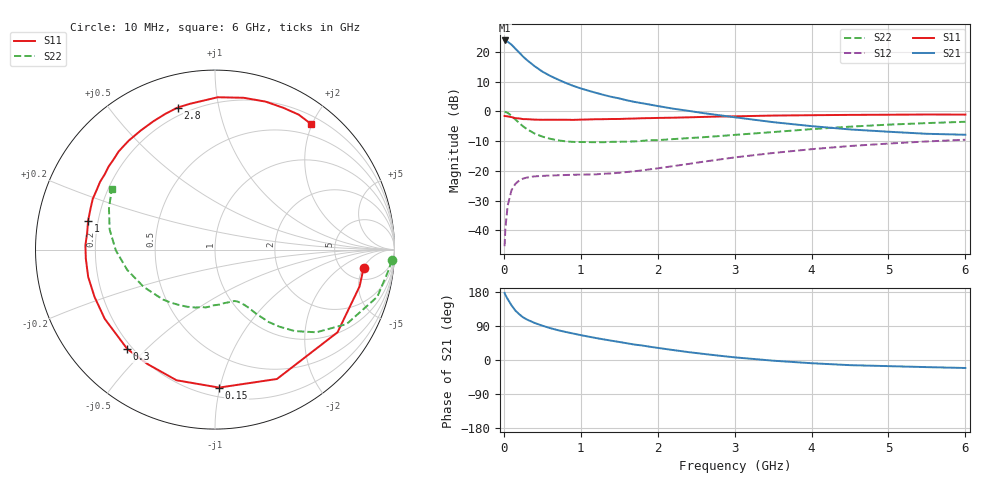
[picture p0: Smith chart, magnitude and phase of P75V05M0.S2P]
! SIEMENS Small Signal Semiconductors
! BFP196
! Si NPN RF Bipolar Junction Transistor in SOT143
! VCE = 5 V  IC = 5 mA
! Common Emitter S-Parameters:  May  1996
# GHz  S  MA  R  50
!  f  S11  S21  S12  S22
! GHz  MAG  ANG  MAG  ANG  MAG  ANG  MAG  ANG
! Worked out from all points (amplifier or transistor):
!   36 points, 10 MHz to 6 GHz, reference 50 ohm
!   highest |S21| = 23.8 dB at 10 MHz (marker M1)
!   |S21| within 3 dB of that: start of sweep to 159.2 MHz
!   unconditionally stable (mu >= 1): 1.146 GHz to 3.193 GHz
!   at 250 MHz: K = 0.25, MSG = 20.5 dB, |S12| = -22.6 dB
!   at 1.4 GHz: K = 1.14, MAG = 10.6 dB, |S12| = -20.9 dB
!   at 6 GHz: K = 0.99, MSG = 0.8 dB, |S12| = -9.6 dB
!   S11 on the Smith chart (normalised r, x): 10 MHz: 7.55, -5.13; 150 MHz: 0.26, -0.99; 300 MHz: 0.18, -0.44; 1 GHz: 0.16, +0.11; 2.8 GHz: 0.16, +0.76; 6 GHz: 0.32, +1.98
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0.01  0.8344 -7.1  15.56 177.0  0.0054 85.8  0.9867 -3.5
0.02  0.8312 -14.3  15.33 171.8  0.0108 84.6  0.9748 -6.6
0.05  0.8236 -34.0  14.78 160.7  0.0261 72.7  0.9419 -16.2
0.1  0.7993 -64.4  13.22 144.2  0.0474 58.5  0.8426 -29.5
0.15  0.7691 -88.3  11.33 130.4  0.0604 47.2  0.7289 -39.2
0.2  0.7589 -106.4  9.73 120.8  0.0687 39.9  0.6356 -45.6
0.25  0.7403 -120.6  8.328 112.7  0.0739 34.3  0.5598 -50.1
0.3  0.7385 -131.5  7.289 106.8  0.077 30.7  0.5029 -53.4
0.4  0.7254 -147.9  5.75 97.8  0.0806 25.9  0.4227 -57.4
0.5  0.7211 -158.6  4.668 90.6  0.0821 23.1  0.3759 -59.8
0.6  0.7228 -167.9  3.963 84.3  0.0832 22.1  0.346 -62.3
0.7  0.7214 -175.9  3.443 78.8  0.0841 21.6  0.3263 -64.7
0.8  0.7224 178.2  3.022 74.2  0.0849 21.6  0.3131 -67.1
1  0.7251 167.1  2.43 65.6  0.0861 23.0  0.3047 -71.6
1.1  0.7298 162.0  2.223 61.7  0.0867 24.2  0.3034 -74.4
1.6  0.7519 142.0  1.532 44.1  0.0954 32.2  0.3095 -90.0
2.2  0.7818 122.0  1.109 26.3  0.1197 39.1  0.3412 -108.9
2.8  0.8184 104.7  0.861 11.4  0.1546 39.7  0.3836 -129.5
3.5  0.8489 89.0  0.658 -1.8  0.1993 34.8  0.4482 -152.3
4.5  0.8714 71.1  0.496 -13.6  0.2611 23.6  0.5525 -179.5
5.5  0.8848 58.2  0.419 -18.8  0.3117 11.0  0.6341 158.7
6  0.881 52.6  0.404 -21.1  0.333 4.3  0.6677 149.4
